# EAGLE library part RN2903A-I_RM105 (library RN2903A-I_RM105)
MICROCHIP - RN2903A-I/RM105 - TRANSCEIVER MODULE, 300KBPS, 928MHZ Source: Datasheet
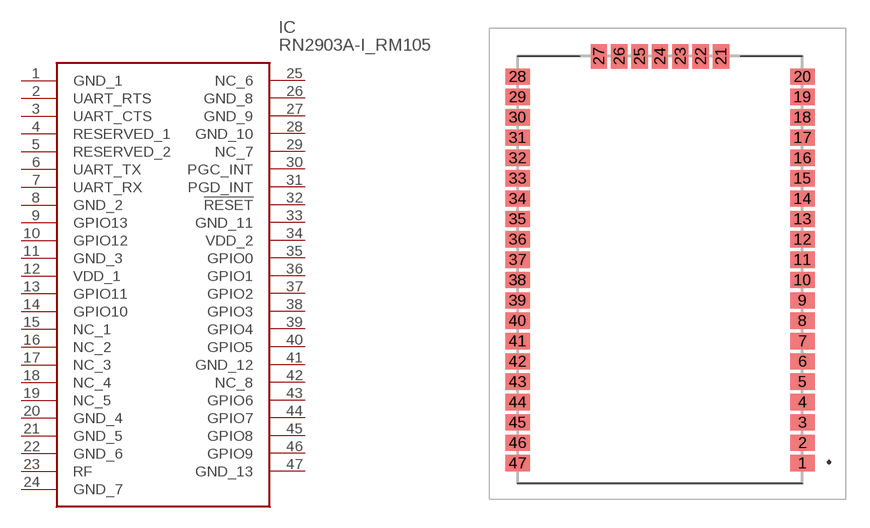
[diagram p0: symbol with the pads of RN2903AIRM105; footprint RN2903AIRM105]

Designator prefix IC

## RN2903A-I_RM105 (Description: MICROCHIP - RN2903A-I/RM105 - TRANSCEIVER MODULE, 300KBPS, 928MHZ; Height: 3.34mm; Manufacturer_Name: Microchip; Manufacturer_Part_Number: RN2903A-I/RM105; Mouser_Part_Number: 579-RN2903A-I/RM105; Mouser_Price-Stock: https://www.mouser.co.uk/ProductDetail/Microchip-Technology/RN2903A-I-RM105?qs=PqoDHHvF648ggy%252BxQbPa3A%3D%3D)  [RN2903AIRM105]
1  GND_1
2  UART_RTS
3  UART_CTS
4  RESERVED_1
5  RESERVED_2
6  UART_TX
7  UART_RX
8  GND_2
9  GPIO13
10  GPIO12
11  GND_3
12  VDD_1
13  GPIO11
14  GPIO10
15  NC_1
16  NC_2
17  NC_3
18  NC_4
19  NC_5
20  GND_4
21  GND_5
22  GND_6
23  RF
24  GND_7
25  NC_6
26  GND_8
27  GND_9
28  GND_10
29  NC_7
30  PGC_INT
31  PGD_INT
32  !RESET
33  GND_11
34  VDD_2
35  GPIO0
36  GPIO1
37  GPIO2
38  GPIO3
39  GPIO4
40  GPIO5
41  GND_12
42  NC_8
43  GPIO6
44  GPIO7
45  GPIO8
46  GPIO9
47  GND_13

## Footprint RN2903AIRM105 (pad centres in mm)
RN2903A-I/RM105-2
smd 1.524 x 1.016: 1 8.89,-12.065; 2 8.89,-10.795; 3 8.89,-9.525; 4 8.89,-8.255; 5 8.89,-6.985; 6 8.89,-5.715; 7 8.89,-4.445; 8 8.89,-3.175; 9 8.89,-1.905; 10 8.89,-0.635; 11 8.89,0.635; 12 8.89,1.905; 13 8.89,3.175; 14 8.89,4.445; 15 8.89,5.715; 16 8.89,6.985; 17 8.89,8.255; 18 8.89,9.525; 19 8.89,10.795; 20 8.89,12.065; 28 -8.89,12.065; 29 -8.89,10.795; 30 -8.89,9.525; 31 -8.89,8.255; 32 -8.89,6.985; 33 -8.89,5.715; 34 -8.89,4.445; 35 -8.89,3.175; 36 -8.89,1.905; 37 -8.89,0.635; 38 -8.89,-0.635; 39 -8.89,-1.905; 40 -8.89,-3.175; 41 -8.89,-4.445; 42 -8.89,-5.715; 43 -8.89,-6.985; 44 -8.89,-8.255; 45 -8.89,-9.525; 46 -8.89,-10.795; 47 -8.89,-12.065
smd 1.016 x 1.524: 21 3.81,13.335; 22 2.54,13.335; 23 1.27,13.335; 24 0,13.335; 25 -1.27,13.335; 26 -2.54,13.335; 27 -3.81,13.335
